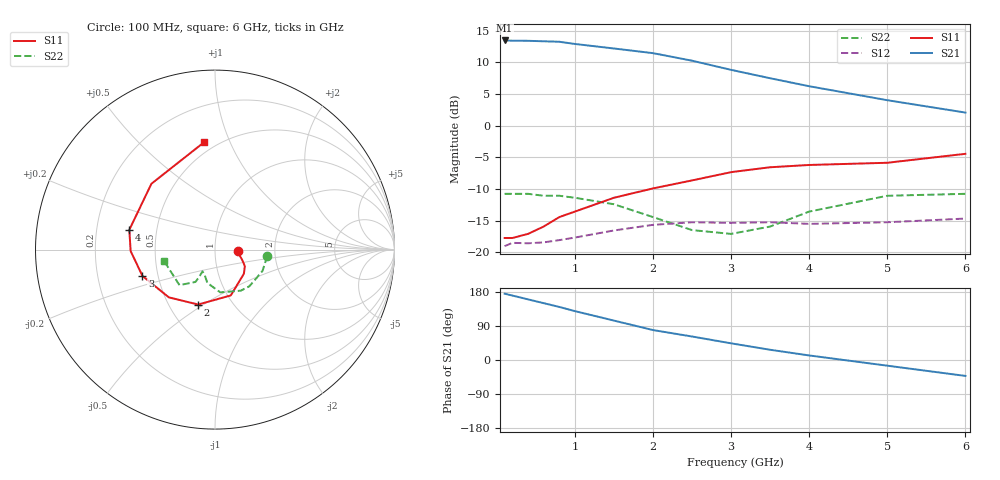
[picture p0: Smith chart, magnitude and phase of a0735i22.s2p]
!  MSA-0735 S AND NOISE PARAMETERS
!  Id=22mA  LAST UPDATED 07-27-92
# ghz s ma r 50
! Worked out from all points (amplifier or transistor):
!   14 points, 100 MHz to 6 GHz, reference 50 ohm
!   highest |S21| = 13.5 dB at 100 MHz (marker M1)
!   |S21| within 3 dB of that: start of sweep to 2.418 GHz
!   unconditionally stable (mu >= 1): start of sweep to 1.81 GHz; 2.615 GHz to end of sweep
!   at 400 MHz: K = 1.13, MAG = 13.8 dB, |S12| = -18.6 dB
!   at 2 GHz: K = 0.98, MSG = 13.6 dB, |S12| = -15.7 dB
!   at 6 GHz: K = 1.20, MAG = 5.7 dB, |S12| = -14.7 dB
!   lowest NFmin = 4.30 dB at 100 MHz
!   S11 on the Smith chart (normalised r, x): 100 MHz: 1.30, -0.02; 2 GHz: 0.70, -0.47; 3 GHz: 0.41, -0.15; 4 GHz: 0.35, +0.10; 6 GHz: 0.43, +0.80
0.1  0.13 -3.0  4.71 175.0  0.112 2.0  0.29 -7.0
0.2  0.13 -6.0  4.69 170.0  0.119 3.0  0.29 -12.0
0.4  0.14 -13.0  4.68 160.0  0.118 6.0  0.29 -24.0
0.6  0.16 -20.0  4.64 150.0  0.12 7.0  0.28 -35.0
0.8  0.19 -29.0  4.6 140.0  0.125 8.0  0.28 -47.0
1  0.21 -40.0  4.42 129.0  0.131 10.0  0.27 -58.0
1.5  0.27 -71.0  4.07 104.0  0.149 10.0  0.24 -83.0
2  0.32 -107.0  3.74 79.0  0.165 7.0  0.19 -103.0
2.5  0.37 -134.0  3.26 62.0  0.173 5.0  0.15 -113.0
3  0.43 -160.0  2.76 44.0  0.171 0.0  0.14 -120.0
3.5  0.47 -179.0  2.37 27.0  0.173 -4.0  0.16 -120.0
4  0.49 167.0  2.05 12.0  0.168 -6.0  0.21 -121.0
5  0.51 134.0  1.59 -15.0  0.173 -11.0  0.28 -135.0
6  0.6 96.0  1.27 -42.0  0.185 -16.0  0.29 -167.0
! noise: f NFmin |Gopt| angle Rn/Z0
0.1  4.3  0.06  1  0.61
0.5  4.4  0.06  4  0.61
1  4.5  0.04  9  0.59
2  5  0.03  -100  0.57
